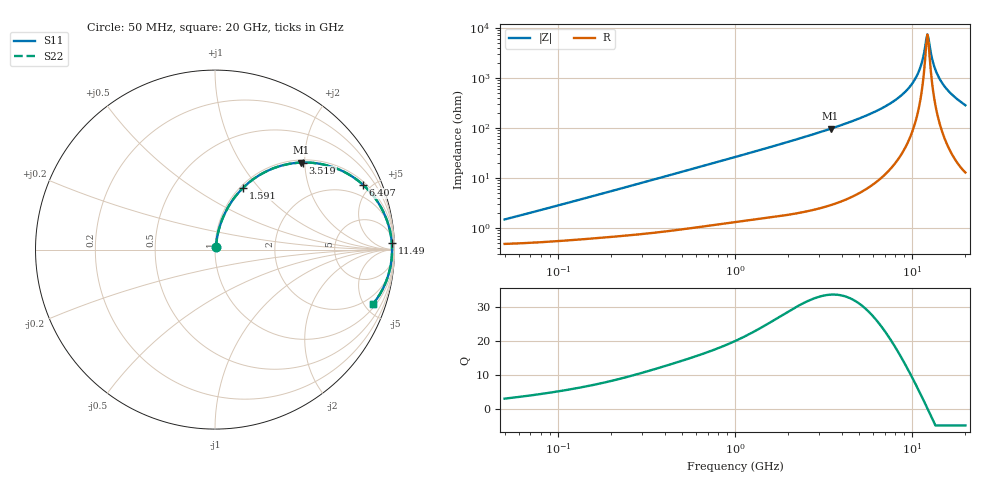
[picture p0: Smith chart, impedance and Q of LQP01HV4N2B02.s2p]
!Murata Part Number: LQP01HV4N2B02
!These Parameters are Measured in Series Mode Connection
!  o--[Z]--o
!Port1  Port2
!  o-------o
!Freq. Start=50[MHz] Stop=20[GHz], 401[Steps]
# Hz S RI R 50
!Freq.(Hz) S11(Real) S11(Imag) S21(Real) S21(Imag) S12(Real) S12(Imag) S22(Real) S22(Imag)
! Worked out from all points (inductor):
!   401 points, 50 MHz to 20 GHz, reference 50 ohm
!   read as one part in series: L = 4.46 nH near 52.3 MHz
!   highest Q = 33.6 at 3.467 GHz (marker M1), where L = 4.42 nH
!   self-resonance near 12.2 GHz
!   S11 on the Smith chart (normalised r, x): 50 MHz: 1.01, +0.03; 1.591 GHz: 1.03, +0.83; 3.519 GHz: 1.06, +1.96; 6.407 GHz: 1.18, +4.49; 11.49 GHz: 16, +45; 20 GHz: 1.26, -5.66
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5e7  0.00499 0.0139  0.995 -0.0139  0.995 -0.0139  0.00499 0.0139
1.364002e8  0.00729 0.0369  0.9927 -0.0369  0.9927 -0.0369  0.00729 0.0369
3.721004e8  0.0177 0.0965  0.9823 -0.0965  0.9823 -0.0965  0.0177 0.0965
1e9  0.0745 0.2386  0.9255 -0.2386  0.9255 -0.2386  0.0745 0.2386
1.590961e9  0.1574 0.3451  0.8426 -0.3451  0.8426 -0.3451  0.1574 0.3451
2.728004e9  0.3546 0.4631  0.6454 -0.4631  0.6454 -0.4631  0.3546 0.4631
3.466789e9  0.4814 0.485  0.5186 -0.485  0.5186 -0.485  0.4814 0.485
3.519108e9  0.4899 0.4853  0.5101 -0.4853  0.5101 -0.4853  0.4899 0.4853
4.748272e9  0.6651 0.4565  0.3349 -0.4565  0.3349 -0.4565  0.6651 0.4565
6.406762e9  0.825 0.3609  0.175 -0.3609  0.175 -0.3609  0.825 0.3609
7.442007e9  0.8889 0.2912  0.1111 -0.2912  0.1111 -0.2912  0.8889 0.2912
8.774992e9  0.942 0.2021  0.058 -0.2021  0.058 -0.2021  0.942 0.2021
9.892087e9  0.9681 0.1314  0.0319 -0.1314  0.0319 -0.1314  0.9681 0.1314
1.082228e10  0.9804 0.0762  0.0196 -0.0762  0.0196 -0.0762  0.9804 0.0762
1.149051e10  0.9849 0.0387  0.0151 -0.0387  0.0151 -0.0387  0.9849 0.0387
1.201863e10  0.9864 0.0103  0.0136 -0.0103  0.0136 -0.0103  0.9864 0.0103
1.220001e10  0.9866 0.00084  0.0134 -0.00084  0.0134 -0.00084  0.9866 0.00084
1.238412e10  0.9865 -0.00867  0.0135 0.00867  0.0135 0.00867  0.9865 -0.00867
1.334722e10  0.9835 -0.0563  0.0165 0.0563  0.0165 0.0563  0.9835 -0.0563
1.460232e10  0.9735 -0.1133  0.0265 0.1133  0.0265 0.1133  0.9735 -0.1133
1.670968e10  0.9451 -0.1974  0.0549 0.1974  0.0549 0.1974  0.9451 -0.1974
2e10  0.8785 -0.3048  0.1215 0.3048  0.1215 0.3048  0.8785 -0.3048
